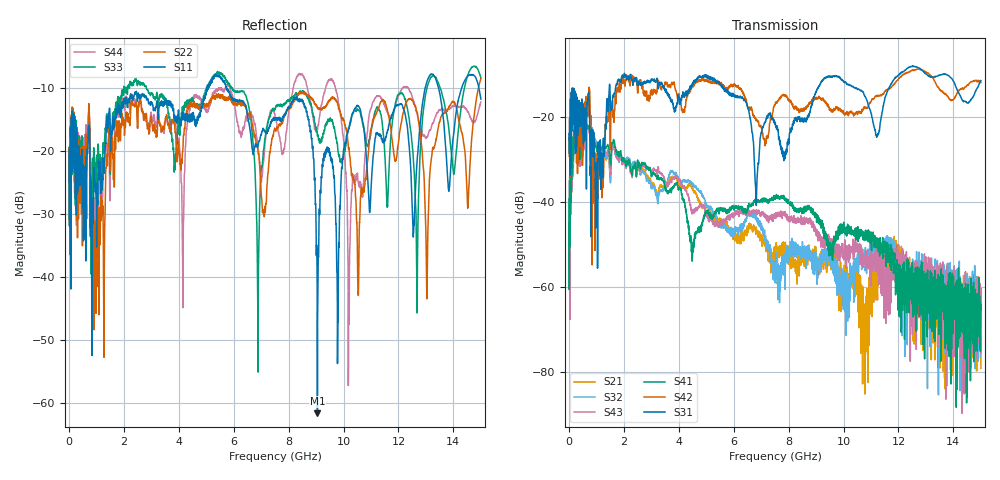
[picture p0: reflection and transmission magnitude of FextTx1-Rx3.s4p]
! FILE: N:\QM 2007\Prüfprotokolle\Highspeed\Konfektionierte Ltg\L45593-D106\D30\8216\0002\Fext\FextTx1-Rx3.s4p
# MHz S RI R 50.00
! FREQ  S11  S12  S13  S14
!  S21  S22  S23  S24
!  S31  S32  S33  S34
!  S41  S42  S43  S44
!  REAL  IMAG  REAL  IMAG  REAL  IMAG  REAL  IMAG
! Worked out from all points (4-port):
!   2999 points, 10 MHz to 15 GHz, reference 50 ohm
!   strongest paths, dB at 10 MHz, 3.755 GHz, 7.505 GHz, 11.26 GHz, 15 GHz:
!     S31: -23.8, -15.9, -21.3, -24.0, -11.4
!     S42: -24.8, -11.8, -17.2, -15.0, -11.8
!     S41: -39.2, -36.6, -39.1, -49.4, -64.2
!     S43: -55.3, -34.8, -42.8, -53.0, -60.8
!     S32: -54.4, -32.6, -55.5, -50.6, -76.2
!     S21: -44.7, -33.9, -52.0, -57.2, -79.1
!   lowest |S11| = -61.6 dB at 9.05 GHz (marker M1), VSWR 1.00, Z = 50.1 + j0.0398 ohm
!   |S11| at or under -10 dB: start of sweep to 5.038 GHz; 5.742 GHz to 12.97 GHz (7.227 GHz wide, 77.2 % of centre); 13.46 GHz to 14.3 GHz (838.1 MHz wide, 6.04 % of centre)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
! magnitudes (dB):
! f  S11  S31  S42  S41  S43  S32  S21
! 10 MHz  -19.8  -23.8  -24.8  -39.2  -55.3  -54.4  -44.7
! 680 MHz  -20.4  -16.4  -19.1  -22.6  -22.8  -22.5  -22.8
! 6.885 GHz  -19.1  -31.1  -21.1  -39.9  -41.9  -44.0  -46.8
! 8.46 GHz  -12.1  -20.8  -18.5  -41.8  -44.0  -51.1  -53.1
! 9.05 GHz  -61.6  -13.4  -15.6  -42.9  -48.1  -56.8  -54.9
! 13.03 GHz  -9.0  -9.9  -9.5  -62.1  -58.0  -59.0  -67.0
! 15 GHz  -11.7  -11.4  -11.8  -64.2  -60.8  -76.2  -79.1
